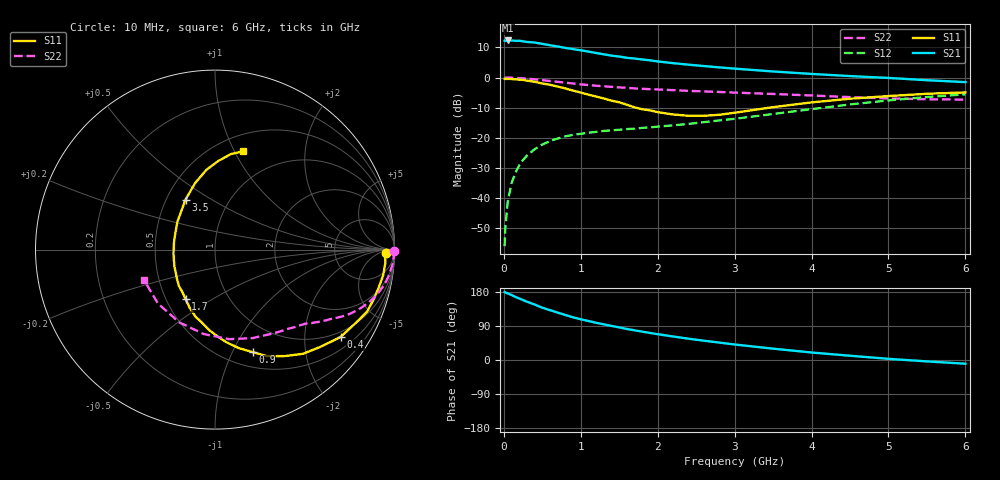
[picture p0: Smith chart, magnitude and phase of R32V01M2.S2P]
! SIEMENS Small Signal Semiconductors
! BFR181
! Si NPN RF Bipolar Junction Transistor in SOT23
! VCE = 2 V  IC = 1.2 mA
! Common Emitter S-Parameters:  May  1996
# GHz  S  MA  R  50
!  f  S11  S21  S12  S22
! GHz  MAG  ANG  MAG  ANG  MAG  ANG  MAG  ANG
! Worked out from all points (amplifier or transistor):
!   36 points, 10 MHz to 6 GHz, reference 50 ohm
!   highest |S21| = 12.3 dB at 50 MHz (marker M1)
!   |S21| within 3 dB of that: start of sweep to 931.9 MHz
!   unconditionally stable (mu >= 1): 1.888 GHz to 3.61 GHz
!   at 250 MHz: K = 0.18, MSG = 19.7 dB, |S12| = -27.3 dB
!   at 1.4 GHz: K = 0.83, MSG = 12.4 dB, |S12| = -17.5 dB
!   at 6 GHz: K = 0.88, MSG = 2.0 dB, |S12| = -5.5 dB
!   S11 on the Smith chart (normalised r, x): 10 MHz: 37, -14; 400 MHz: 0.84, -2.98; 900 MHz: 0.66, -1.20; 1.7 GHz: 0.63, -0.39; 3.5 GHz: 0.62, +0.39; 6 GHz: 0.67, +1.08
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0.01  0.9538 -1.0  4.098 179.4  0.0016 88.6  0.9986 -0.4
0.02  0.9481 -1.7  4.035 178.1  0.0033 91.3  0.9961 -0.9
0.05  0.9524 -4.3  4.133 175.7  0.0086 87.2  0.9966 -2.1
0.1  0.9475 -8.8  4.129 171.6  0.0177 84.7  0.9953 -4.2
0.15  0.9356 -13.4  4.068 166.3  0.0264 81.2  0.9865 -6.3
0.2  0.9259 -17.6  4.084 162.3  0.0349 78.5  0.9801 -8.3
0.3  0.891 -26.3  3.902 153.8  0.0509 73.5  0.961 -12.0
0.4  0.8527 -34.8  3.82 146.4  0.0648 68.8  0.9364 -15.6
0.5  0.7991 -42.7  3.629 137.9  0.0776 64.4  0.9071 -18.8
0.6  0.76 -49.8  3.443 131.5  0.0887 60.5  0.879 -21.5
0.7  0.7103 -56.6  3.282 125.0  0.0976 57.4  0.8513 -23.9
0.9  0.608 -69.9  2.97 112.6  0.1123 52.3  0.7978 -27.9
1.1  0.5208 -82.9  2.698 102.8  0.1218 48.9  0.751 -31.0
1.4  0.4147 -99.9  2.316 89.9  0.1333 46.1  0.7028 -35.0
1.7  0.321 -120.6  2.069 78.3  0.1424 46.0  0.6617 -38.2
1.9  0.2859 -134.7  1.934 71.4  0.1497 46.6  0.6428 -40.5
2.2  0.2445 -157.9  1.738 62.0  0.1615 47.7  0.6195 -44.2
2.8  0.2417 155.2  1.478 46.0  0.1949 51.0  0.5778 -52.8
3.5  0.3236 120.5  1.264 29.9  0.2493 51.5  0.5358 -67.0
4.5  0.4468 96.2  1.06 11.2  0.3586 45.7  0.4746 -97.6
5.5  0.5393 80.6  0.905 -3.7  0.476 33.2  0.4375 -136.5
6  0.5683 74.3  0.842 -9.8  0.5282 25.5  0.4312 -157.0
